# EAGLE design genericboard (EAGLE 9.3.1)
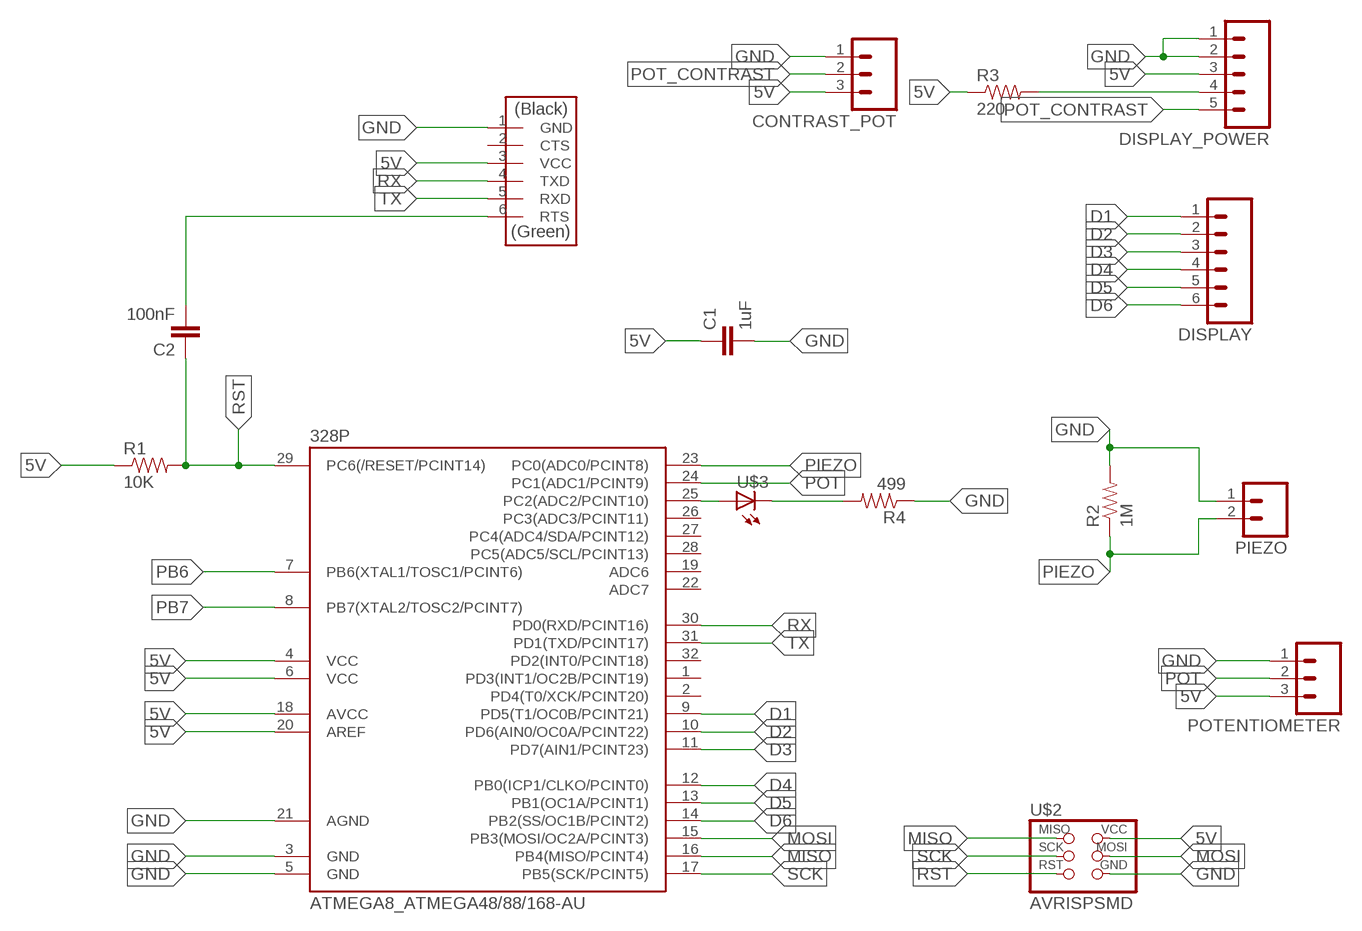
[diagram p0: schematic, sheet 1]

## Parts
328P  ATMEGA8_ATMEGA48/88/168-AU  [ATMEGA8_TQFP32-08]
C1  1uF  01_SPARKFUN_CAP1206  [01_SPARKFUN_1206]
C2  100nF  01_SPARKFUN_CAP1206  [01_SPARKFUN_1206]
CONTRAST_POT  M03  [03P]
DISPLAY  M06  [06P]
DISPLAY_POWER  M05  [05P]
FTDI  FTDI-SMD-HEADER  [1X06SMD]
PIEZO  M02  [02P]
POTENTIOMETER  M03  [03P]
R1  10K  01_SPARKFUN_RESISTOR1206  [01_SPARKFUN_1206]
R2  1M  01_SPARKFUN_RESISTOR1206  [01_SPARKFUN_1206]
R3  220  01_SPARKFUN_RESISTOR1206  [01_SPARKFUN_1206]
R4  499  01_SPARKFUN_RESISTOR1206  [01_SPARKFUN_1206]
U$2  AVRISPSMD  [2X03SMD]
U$3  01_FAB_HELLO_LED1206  [01_FAB_HELLO_1206]

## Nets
5V: 328P.4(VCC) 328P.6(VCC) 328P.18(AVCC) 328P.20(AREF) C1.1 CONTRAST_POT.3 DISPLAY_POWER.3 FTDI.3(VCC) POTENTIOMETER.3 R1.1 R3.1 U$2.2(VCC)
D1: 328P.9(PD5(T1/OC0B/PCINT21)) DISPLAY.1
D2: 328P.10(PD6(AIN0/OC0A/PCINT22)) DISPLAY.2
D3: 328P.11(PD7(AIN1/PCINT23)) DISPLAY.3
D4: 328P.12(PB0(ICP1/CLKO/PCINT0)) DISPLAY.4
D5: 328P.13(PB1(OC1A/PCINT1)) DISPLAY.5
D6: 328P.14(PB2(SS/OC1B/PCINT2)) DISPLAY.6
GND: 328P.3(GND) 328P.5(GND) 328P.21(AGND) C1.2 CONTRAST_POT.1 DISPLAY_POWER.1 DISPLAY_POWER.2 FTDI.1(GND) PIEZO.1 POTENTIOMETER.1 R2.2 R4.1 U$2.6(GND)
MISO: 328P.16(PB4(MISO/PCINT4)) U$2.1(MISO)
MOSI: 328P.15(PB3(MOSI/OC2A/PCINT3)) U$2.4(MOSI)
N$1: C2.2 FTDI.6(RTS)
N$2: DISPLAY_POWER.4 R3.2
N$3: 328P.25(PC2(ADC2/PCINT10)) U$3.1(A)
N$4: R4.2 U$3.2(C)
PB6: 328P.7(PB6(XTAL1/TOSC1/PCINT6))
PB7: 328P.8(PB7(XTAL2/TOSC2/PCINT7))
PIEZO: 328P.23(PC0(ADC0/PCINT8)) PIEZO.2 R2.1
POT: 328P.24(PC1(ADC1/PCINT9)) POTENTIOMETER.2
POT_CONTRAST: CONTRAST_POT.2 DISPLAY_POWER.5
RST: 328P.29(PC6(/RESET/PCINT14)) C2.1 R1.2 U$2.5(RST)
RX: 328P.30(PD0(RXD/PCINT16)) FTDI.4(TXD)
SCK: 328P.17(PB5(SCK/PCINT5)) U$2.3(SCK)
TX: 328P.31(PD1(TXD/PCINT17)) FTDI.5(RXD)
Unconnected: 328P.1(PD3(INT1/OC2B/PCINT19)) 328P.2(PD4(T0/XCK/PCINT20)) 328P.19(ADC6) 328P.22(ADC7) 328P.26(PC3(ADC3/PCINT11)) 328P.27(PC4(ADC4/SDA/PCINT12)) 328P.28(PC5(ADC5/SCL/PCINT13)) 328P.32(PD2(INT0/PCINT18)) FTDI.2(CTS)

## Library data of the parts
328P = satshakit_cnc:ATMEGA8_ATMEGA48/88/168
C1 C2 = satshakit_cnc:01_SPARKFUN_CAP: Capacitor
CONTRAST_POT POTENTIOMETER = con-amp-quick:M03: AMP QUICK CONNECTOR; OC_FARNELL: unknown; OC_NEWARK: unknown
DISPLAY = con-amp-quick:M06: AMP QUICK CONNECTOR; OC_FARNELL: unknown; OC_NEWARK: unknown
DISPLAY_POWER = con-amp-quick:M05: AMP QUICK CONNECTOR; OC_FARNELL: unknown; OC_NEWARK: unknown
FTDI = fab:FTDI-SMD-HEADER
PIEZO = con-amp-quick:M02: AMP QUICK CONNECTOR; OC_FARNELL: unknown; OC_NEWARK: unknown
R1-R4 = satshakit_cnc:01_SPARKFUN_RESISTOR: Resistor
U$2 = fab:AVRISP
U$3 = satshakit_cnc:01_FAB_HELLO_LED

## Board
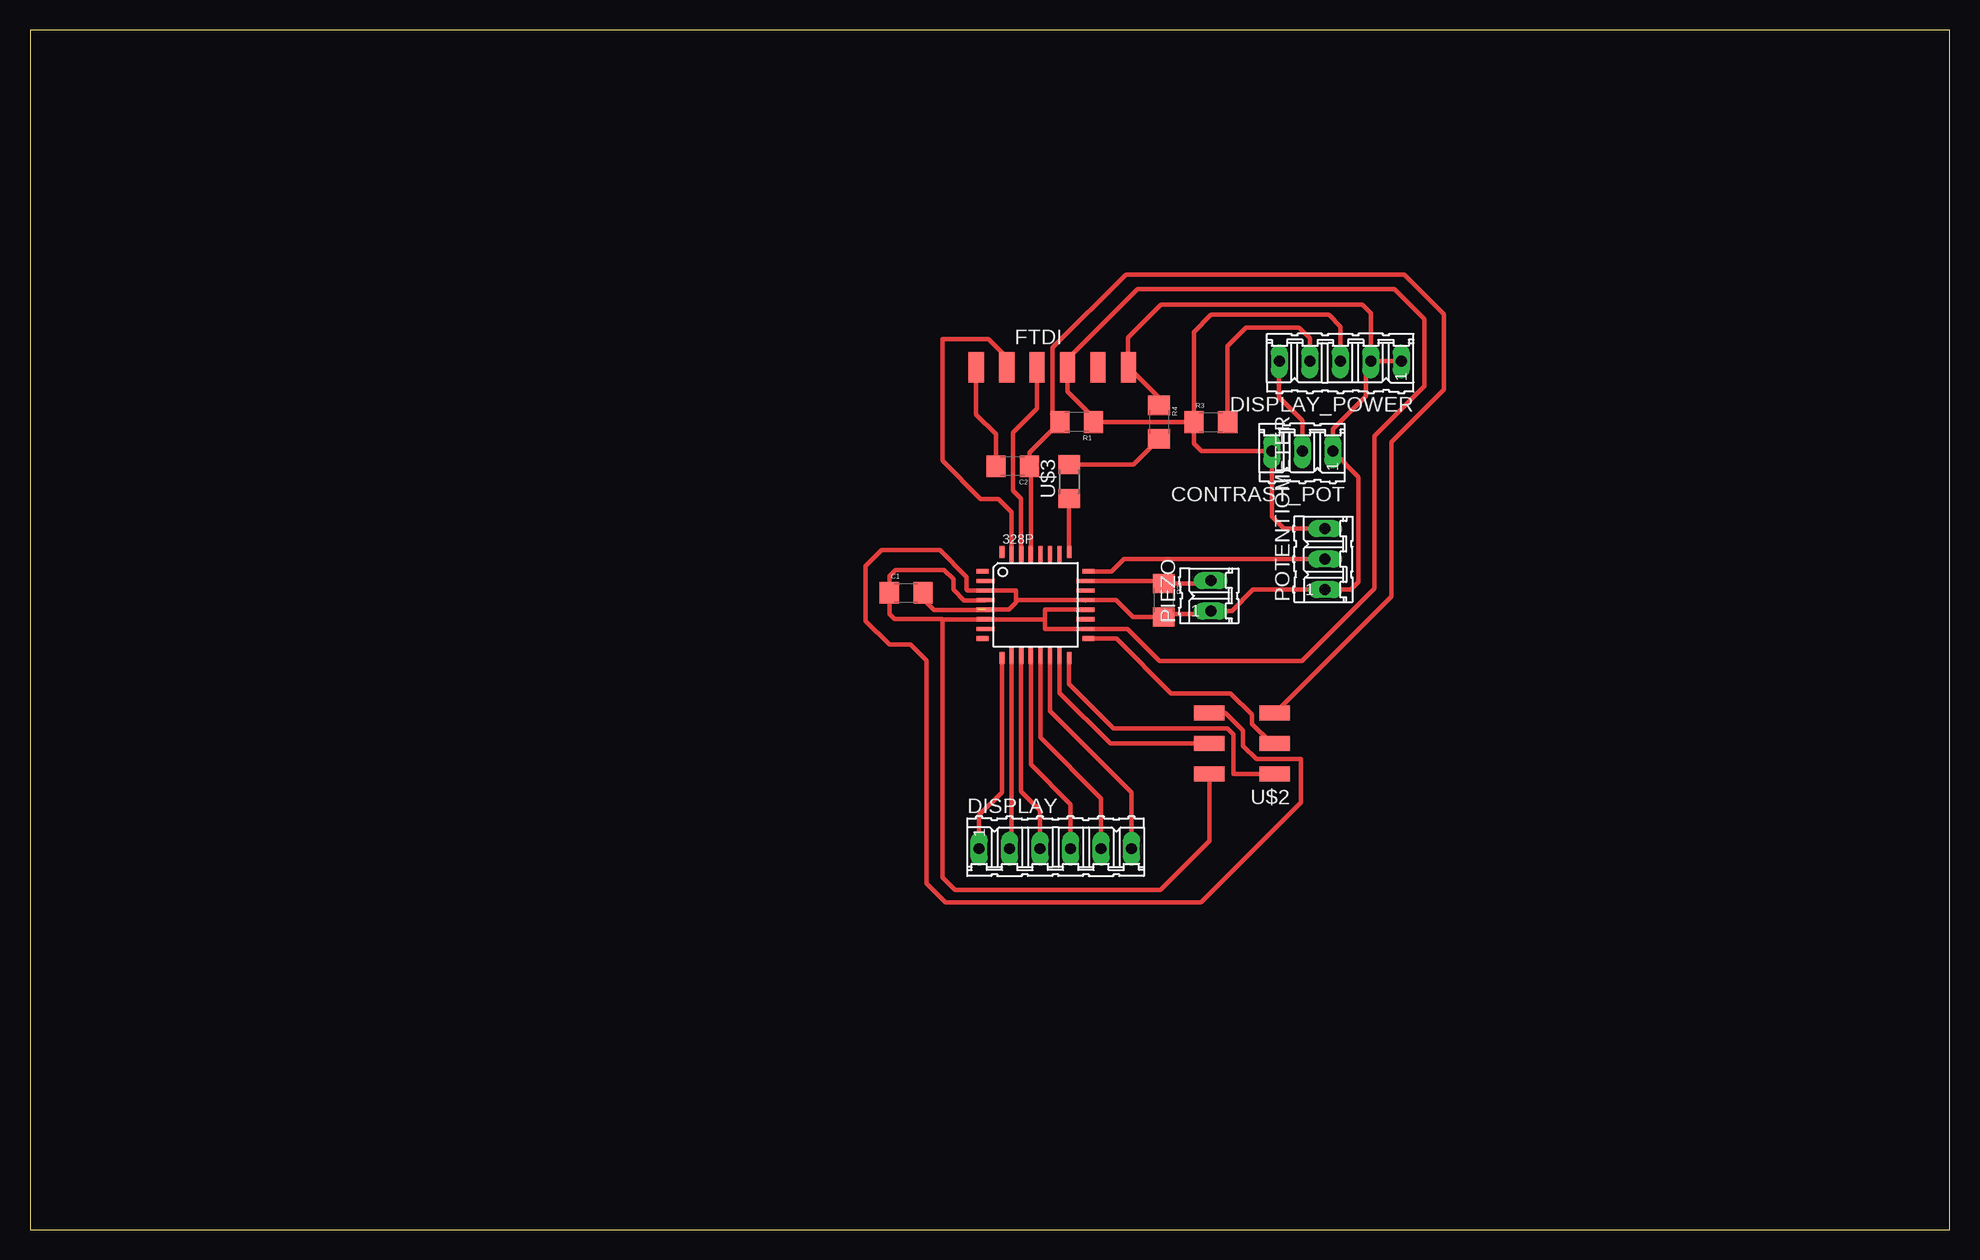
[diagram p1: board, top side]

Size 160 x 100 mm. Coordinates in mm from the lower left corner, seen from the top.
Outline: 0,0 160,0 160,100 0,100 0,0
Copper layers (1*16): Top 0.035mm / dielectric 1.5mm / Bottom 0.035mm
Design rules "default *": minimum track width 6mil, minimum drill 0.35mm, track to track 17mil, track to pad 17mil, pad to pad 17mil, via to via 17mil, smd to smd 17mil, copper to edge 40mil, drill to drill 6mil, minimum pad ring 10mil, minimum via ring 8mil, stop-mask expansion 4mil, vias tented up to drill 0mil, thermal gap 10mil

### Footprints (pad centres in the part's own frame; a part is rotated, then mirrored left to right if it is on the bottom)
ATMEGA8_TQFP32-08 = smd 1.016 x 0.406: 1 -4.42,2.8; 8 -4.42,-2.8; 17 4.42,-2.8; 24 4.42,2.8 | smd 1.524 x 0.356: 2 -4.166,2; 3 -4.166,1.2; 4 -4.166,0.4; 5 -4.166,-0.4; 6 -4.166,-1.2; 7 -4.166,-2; 18 4.166,-2; 19 4.166,-1.2; 20 4.166,-0.4; 21 4.166,0.4; 22 4.166,1.2; 23 4.166,2 | smd 0.406 x 1.016: 9 -2.8,-4.42; 16 2.8,-4.42; 25 2.8,4.42; 32 -2.8,4.42 | smd 0.356 x 1.524: 10 -2,-4.166; 11 -1.2,-4.166; 12 -0.4,-4.166; 13 0.4,-4.166; 14 1.2,-4.166; 15 2,-4.166; 26 2,4.166; 27 1.2,4.166; 28 0.4,4.166; 29 -0.4,4.166; 30 -1.2,4.166; 31 -2,4.166
01_SPARKFUN_1206 = smd 1.6 x 1.8: 1 -1.4,0; 2 1.4,0
03P = drill 0.914 long: 1 -2.54,0; 2 0,0; 3 2.54,0
06P = drill 0.914 long: 1 -6.35,0; 2 -3.81,0; 3 -1.27,0; 4 1.27,0; 5 3.81,0; 6 6.35,0
05P = drill 0.914 long: 1 -5.08,0; 2 -2.54,0; 3 0,0; 4 2.54,0; 5 5.08,0
1X06SMD = smd 2.54 x 1.27: 1 0,6.35; 2 0,3.81; 3 0,1.27; 4 0,-1.27; 5 0,-3.81; 6 0,-6.35
02P = drill 0.914 long: 1 -1.27,0; 2 1.27,0
2X03SMD = smd 2.54 x 1.27: 1 -2.54,2.54; 2 2.92,2.54; 3 -2.54,0; 4 2.92,0; 5 -2.54,-2.54; 6 2.92,-2.54
01_FAB_HELLO_1206 = smd 1.6 x 1.803: 1 -1.422,0; 2 1.422,0

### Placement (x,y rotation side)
328P  83.82,52.07 0 top
C1  73.03,53.09 0 top
C2  81.92,63.63 180 top
CONTRAST_POT  106.05,64.9 180 top
DISPLAY  85.47,31.75 0 top
DISPLAY_POWER  109.22,72.39 180 top
FTDI  85.22,71.88 270 top
PIEZO  98.42,52.83 90 top
POTENTIOMETER  107.95,55.88 90 top
R1  87.25,67.31 180 top
R2  94.49,52.45 270 top
R3  98.42,67.31 0 top
R4  94.11,67.31 270 top
U$2  101.22,40.51 180 top
U$3  86.61,62.36 90 top

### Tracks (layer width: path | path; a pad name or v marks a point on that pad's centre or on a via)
5V
  Top 0.356: U$2.2 98.3,32.39 94.23,28.32 77.09,28.32 76.07,29.34 76.07,50.87 | 79.67,50.88 328P.6 | 328P.4 79.64,52.46 78.64,52.46 78.64,52.45 77.85,52.45 76.96,53.34 76.96,54.23 76.2,54.99 72.14,54.99 71.62,54.48 C1.1 71.62,51.31 72.06,50.88 76.02,50.88 76.02,50.87 76.07,50.87 | 328P.6 76.07,50.87 | R3.1 R1.1 88.65,67.69 86.49,69.85 FTDI.3 86.49,72.57 92.3,78.38 113.74,78.38 116.23,75.89 116.23,70.31 112.06,66.14 112.06,53.44 106.02,47.4 94.13,47.4 91.46,50.07 328P.18 84.62,50.07 84.62,50.87 | CONTRAST_POT.3 103.38,64.9 | 103.38,64.9 97.66,64.9 97.03,65.53 R3.1 | POTENTIOMETER.3 104.52,58.42 103.5,59.44 103.5,64.77 103.38,64.9 | DISPLAY_POWER.3 109.22,75.29 108.25,76.25 98.45,76.25 97.03,74.83 R3.1 | 84.62,50.87 328P.6 | 84.62,50.87 84.62,51.67 328P.20
D1
  Top 0.356: DISPLAY.1 79.12,34.54 81.02,36.44 328P.9
D2
  Top 0.356: 81.79,31.88 DISPLAY.2 81.82,31.91 328P.10
D3
  Top 0.356: 328P.11 82.62,36.51 84.2,34.92 DISPLAY.3
D4
  Top 0.356: 328P.12 83.42,38.75 86.74,35.43 DISPLAY.4
D5
  Top 0.356: 328P.13 84.22,41 89.28,35.94 DISPLAY.5
D6
  Top 0.356: 328P.14 85.02,43.25 91.82,36.45 DISPLAY.6
GND  (1 unrouted)
  Top 0.356: 87.97,52.46 328P.21 | 108.08,53.21 POTENTIOMETER.1 | 328P.21 90.53,52.47 91.95,51.05 R2.2 94.74,51.3 98.17,51.3 PIEZO.1 100.18,51.56 101.96,53.34 POTENTIOMETER.1 | 78.97,51.67 78.96,51.67 75.34,51.67 74.42,52.58 C1.2 | POTENTIOMETER.1 110.11,53.34 110.74,53.98 110.74,62.74 CONTRAST_POT.1 108.58,66.73 111.35,69.49 111.35,71.98 DISPLAY_POWER.2 | R4.1 94.11,69.34 FTDI.1 91.54,71.91 91.54,74.37 94.28,77.11 111.05,77.11 111.76,76.4 DISPLAY_POWER.2 | DISPLAY_POWER.2 DISPLAY_POWER.1 | 328P.5 81.59,51.67 82.19,52.27 82.19,52.32 | 82.19,52.32 82.19,53.27 328P.3 78.15,53.26 78.08,53.34 78.08,54.41 75.84,56.64 70.97,56.64 69.65,55.32 69.65,50.75 71.63,48.77 73.41,48.77 74.73,47.45 74.73,28.85 76.3,27.28 97.59,27.28 105.92,35.61 105.92,39.22 102.21,39.22 101.12,40.31 101.12,41.6 99.67,43.05 U$2.6 | 328P.21 82.34,52.47 82.19,52.32
MISO
  Top 0.356: 328P.16 86.62,45.46 90.3,41.78 99.82,41.78 100.33,41.27 100.33,37.97 102.49,37.97 102.62,37.97 U$2.1
MOSI
  Top 0.356: 328P.15 85.82,44.74 90.04,40.51 U$2.4
N$1
  Top 0.356: C2.2 80.52,66.3 78.87,67.94 FTDI.6
N$2
  Top 0.356: R3.2 99.83,73.66 101.35,75.18 105.79,75.18 106.68,74.3 DISPLAY_POWER.4
N$3
  Top 0.356: 328P.25 U$3.1
N$4
  Top 0.356: U$3.2 91.98,63.78 R4.2
PIEZO
  Top 0.356: PIEZO.2 98.17,53.85 R2.1 94.27,54.07 328P.23
POT
  Top 0.356: POTENTIOMETER.2 91.19,55.88 90.16,54.86 88.25,54.86 328P.24
POT_CONTRAST
  Top 0.356: CONTRAST_POT.2 106.05,67.44 104.09,69.39 104.09,72.34 DISPLAY_POWER.5
RST
  Top 0.356: 328P.29 83.42,63.52 C2.1 83.31,64.78 R1.2 | U$2.5 113.49,52.78 113.49,65.63 117.86,70 117.86,76.3 114.55,79.6 91.34,79.6 85.24,73.51 85.24,67.92 R1.2 | 85.19,67.97 R1.2
RX
  Top 0.356: 328P.30 82.62,60.94 81.94,61.62 81.94,66.45 83.95,68.45 FTDI.4
SCK
  Top 0.356: 328P.17 90.56,49.27 95.12,44.7 100.08,44.7 101.85,42.93 101.85,42.16 103.38,40.64 103.38,40.51 | 103.12,40.51 103.38,40.51 | 103.38,40.51 U$2.3
TX
  Top 0.356: 328P.31 81.82,59.81 80.72,60.91 79.25,60.91 76.05,64.11 76.05,74.22 79.91,74.22 81.43,72.69 81.41,72.67 FTDI.5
